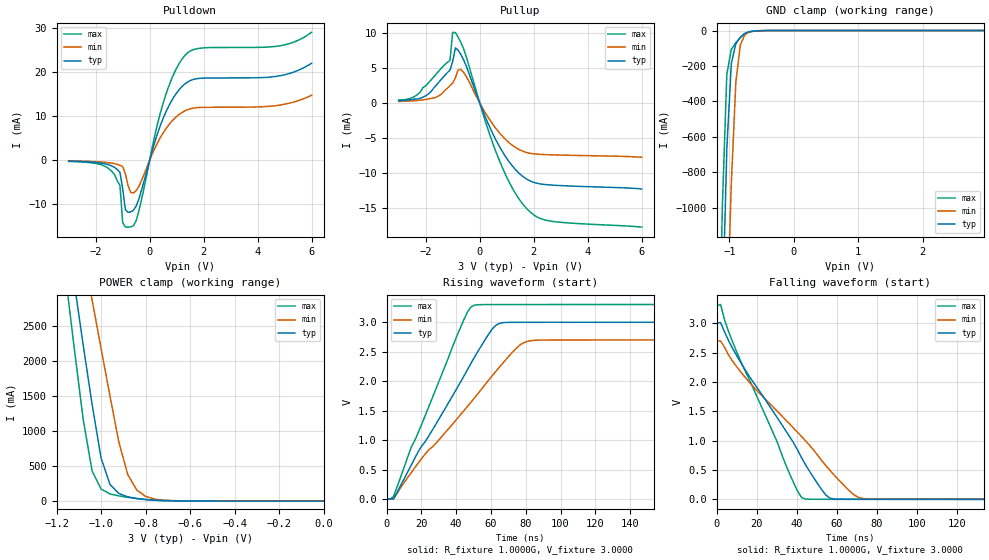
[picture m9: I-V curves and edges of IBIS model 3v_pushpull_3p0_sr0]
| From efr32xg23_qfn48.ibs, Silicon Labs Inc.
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|   Model 3v_pushpull_3p0_sr0
[Model]  3v_pushpull_3p0_sr0
Model_type 3-state
Polarity   Non-Inverting
Enable   Active-High
C_comp   1.6300pF   1.4000pF   2.7000pF
[Temperature Range]   25.0000   0.1250k   -40.0000
[Pullup Reference]   3.0000V   2.7000V   3.3000V
[Pulldown Reference]   0.0V   0.0V   0.0V
[POWER Clamp Reference]   3.0000V   2.7000V   3.3000V
[GND Clamp Reference]   0.0V   0.0V   0.0V
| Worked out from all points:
|   slope of the pulldown table from 0 to 0.45 V, typ, clamps not added: 51.6 ohm
|   slope of the pullup table from 0 to 0.45 V, typ, clamps not added: 109 ohm
|   GND clamp passes 1 mA (typ) near -0.52 V on its own axis
|   POWER clamp passes 1 mA (typ) near -0.53 V on its own axis
|   rising waveform, R_fixture 1.0000G, V_fixture 3.0000: 20-80 % time 35.8ns typ, 46.2ns min, 27.2ns max; typ from 0 V to 3 V
|   falling waveform, R_fixture 1.0000G, V_fixture 3.0000: 20-80 % time 33.3ns typ, 43.1ns min, 25.2ns max; typ from 3 V to 0 V
[Pulldown]
|Voltage   I(typ)   I(min)   I(max)
-3V       -196.9uA   -139.6uA   -248uA
-1.4V     -1.296mA   -652.3uA   -2.541mA
-1.1V     -2.73mA    -1.142mA   -5.692mA
-1V       -6.397mA   -1.401mA   -14.08mA
-900mV    -11.14mA   -3.027mA   -15.11mA
-700mV    -11.68mA   -7.305mA   -15.07mA
-600mV    -11.31mA   -7.41mA    -14.81mA
-400mV    -8.771mA   -5.91mA    -11.48mA
500mV     9.508mA    6.206mA    12.93mA
1.3V      17.26mA    11.17mA    23.71mA
4.9V      19.23mA    12.58mA    26.01mA
6V        21.97mA    14.71mA    28.97mA
[Pullup]
|Voltage   I(typ)   I(min)   I(max)
-3V       282.4uA    190uA      390.9uA
-2V       984.3uA    472.1uA    2.405mA
-1.1V     4.67mA     2.452mA    6.037mA
-1V       5.874mA    2.805mA    10.08mA
-900mV    7.854mA    3.538mA    10.04mA
-800mV    7.546mA    4.682mA    9.417mA
-600mV    6.183mA    4.393mA    7.771mA
700mV     -6.032mA   -4.156mA   -7.968mA
1.3V      -9.453mA   -6.326mA   -12.81mA
1.8V      -11.05mA   -7.178mA   -15.38mA
2.7V      -11.79mA   -7.457mA   -16.98mA
6V        -12.34mA   -7.803mA   -17.81mA
[GND_clamp]
|Voltage   I(typ)   I(min)   I(max)
-3V       -32.58A    -30.59A    -34.3A
-1.18V    -2.82A     -3.643A    -2.261A
-1.11V    -1.644A    -2.575A    -1.001A
-1.04V    -666.4mA   -1.673A    -246.5mA
-970mV    -186.7mA   -861.8mA   -106.7mA
-900mV    -73.86mA   -290.7mA   -68.98mA
-830mV    -38.01mA   -80.48mA   -39.62mA
-760mV    -15.97mA   -23.02mA   -17.36mA
-690mV    -6.612mA   -7.853mA   -7.292mA
-410mV    -117.4uA   -298.1uA   -56.99uA
2.95V     978pA      6.282uA    846.4pA
[POWER_clamp]
|Voltage   I(typ)   I(min)   I(max)
-3V       48.87A     43.6A      53.88A
-1.16V    4.025A     5.101A     3.218A
-1.12V    3.102A     4.315A     2.168A
-1.08V    2.218A     3.569A     1.158A
-1.04V    1.372A     2.862A     425.9mA
-1V       614.1mA    2.175A     173.1mA
-960mV    237.5mA    1.499A     101.5mA
-920mV    109mA      838.4mA    74.91mA
-880mV    61.26mA    377.1mA    54.02mA
-840mV    37.84mA    159.1mA    37.05mA
-720mV    7.412mA    13.58mA    7.87mA
0V        1.019nA    10.64nA    1.026nA
[Ramp]
| variable   typ   min   max
dV/dt_r  1.7814/38.3546n   1.5945/50.2711n   1.9647/28.7094n
dV/dt_f  1.7920/36.5175n   1.6079/48.7486n   1.9737/26.8576n
R_load = 10.0000k
[Rising Waveform]
R_fixture= 1.0000G
V_fixture= 3.0000
V_fixture_min= 2.7000
V_fixture_max= 3.3000
|time   V(typ)   V(min)   V(max)
0s        20.01uV    58.89uV    8.402uV
4.04ns    9.374mV    849.3uV    49.91mV
14.14ns   574.9mV    448.5mV    876mV
20.2ns    903mV      690.3mV    1.271V
42.42ns   1.981V     1.43V      2.905V
48.48ns   2.302V     1.643V     3.257V
62.63ns   2.944V     2.161V     3.299V
74.75ns   2.998V     2.564V     3.299V
80.81ns   2.999V     2.674V     3.299V
200ns     3V         2.7V       3.3V
[Falling Waveform]
R_fixture= 1.0000G
V_fixture= 3.0000
V_fixture_min= 2.7000
V_fixture_max= 3.3000
|time   V(typ)   V(min)   V(max)
0s        3V         2.7V       3.3V
2.02ns    3.011V     2.699V     3.319V
4.04ns    2.849V     2.588V     3.053V
10.1ns    2.446V     2.256V     2.509V
42.42ns   708.9mV    1.07V      31.14mV
52.53ns   163mV      659.1mV    762uV
56.57ns   20.9mV     494.8mV    550.4uV
66.67ns   1.27mV     132.7mV    336.5uV
72.73ns   788.4uV    14.61mV    274.7uV
200ns     20.29uV    60.32uV    8.537uV
